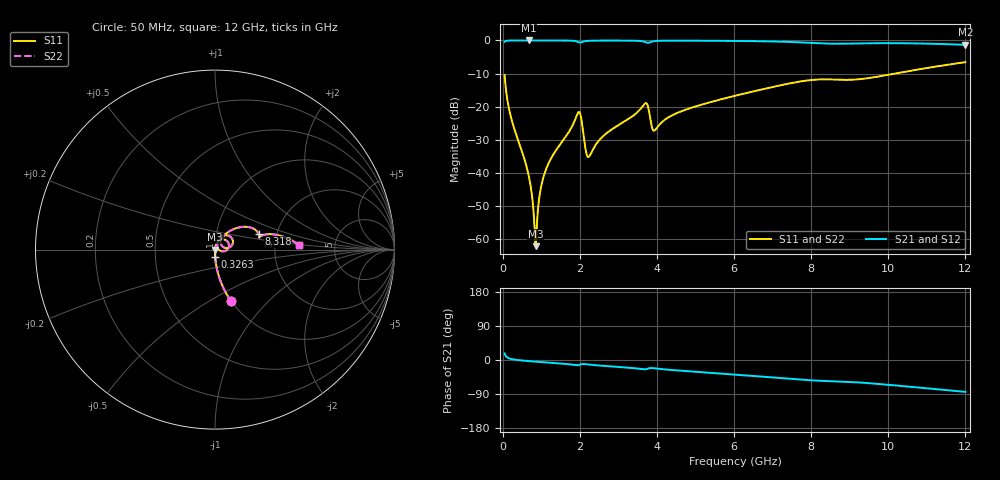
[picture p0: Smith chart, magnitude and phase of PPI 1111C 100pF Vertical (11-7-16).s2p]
# GHz S MA R 50
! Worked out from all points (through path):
!   1601 points, 50 MHz to 12 GHz, reference 50 ohm
!   highest |S21| = -0.01 dB at 669.9 MHz (marker M1); lowest = -1.3 dB at 12 GHz (marker M2)
!   group delay of S21, straight-line fit = 19.3 ps
!   lowest |S11| = -62.1 dB at 856.6 MHz (marker M3), VSWR 1.00, Z = 50.1 + j0.00533 ohm
!   |S11| at or under -10 dB: start of sweep to 10.18 GHz
!   |S22| runs from -62.1 to -6.6 dB; largest |S21 - S12| = 0
!   S11 on the Smith chart (normalised r, x): 50 MHz: 1.00, -0.63; 326.3 MHz: 1.00, -0.08; 8.318 GHz: 1.61, +0.30; 12 GHz: 2.76, +0.18
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0.05  0.3013 -72.7  0.9533 17.3  0.9533 17.3  0.3013 -72.7
0.1769688  0.08556 -85.7  0.9959 4.0  0.9959 4.0  0.08556 -85.7
0.3263437  0.0417 -88.6  0.9986 0.7  0.9986 0.7  0.0417 -88.6
0.6699063  0.009382 -88.7  0.9992 -2.9  0.9992 -2.9  0.009382 -88.7
0.8192812  0.001783 -69.0  0.9992 -4.1  0.9992 -4.1  0.001783 -69.0
0.856625  0.000785 3.9  0.9992 -4.4  0.9992 -4.4  0.000785 3.9
0.9985312  0.006287 76.7  0.9991 -5.5  0.9991 -5.5  0.006287 76.7
1.170313  0.01319 78.9  0.9988 -6.8  0.9988 -6.8  0.01319 78.9
1.939594  0.07773 45.1  0.9575 -13.8  0.9575 -13.8  0.07773 45.1
2.044156  0.06278 -4.0  0.9375 -10.9  0.9375 -10.9  0.06278 -4.0
2.156188  0.02178 -2.0  0.9784 -11.2  0.9784 -11.2  0.02178 -2.0
2.230875  0.01746 31.2  0.9871 -12.1  0.9871 -12.1  0.01746 31.2
2.611781  0.03624 67.9  0.995 -15.4  0.995 -15.4  0.03624 67.9
3.687281  0.1112 41.7  0.9498 -24.6  0.9498 -24.6  0.1112 41.7
3.903875  0.04403 27.0  0.9702 -21.7  0.9702 -21.7  0.04403 27.0
4.038312  0.05117 52.8  0.9862 -23.3  0.9862 -23.3  0.05117 52.8
4.598469  0.08371 58.9  0.9917 -28.0  0.9917 -28.0  0.08371 58.9
6.025  0.146 49.1  0.9828 -38.5  0.9828 -38.5  0.146 49.1
8.019156  0.2532 24.7  0.9174 -53.7  0.9174 -53.7  0.2532 24.7
8.317906  0.2587 19.7  0.9003 -55.1  0.9003 -55.1  0.2587 19.7
10.01331  0.304 16.3  0.9103 -65.6  0.9103 -65.6  0.304 16.3
12  0.4697 3.0  0.8596 -84.2  0.8596 -84.2  0.4697 3.0
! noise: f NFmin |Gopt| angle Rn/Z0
0.05  0.0003497  0.8581  0.4698  0.0005274
1.372  0.004157  0.701  6.968  0.002714
2.701  0.009886  0.7479  13.71  0.007782
4.031  0.02179  0.8245  20.4  0.02526
5.36  0.01492  0.6904  26.47  0.008901
6.682  0.02513  0.7664  32.83  0.02017
8.012  0.06096  0.8805  39.17  0.09808
9.341  0.07245  0.8861  45.05  0.1179
10.67  0.05495  0.8386  50.45  0.05907
12  0.04955  0.8095  55.48  0.04258
